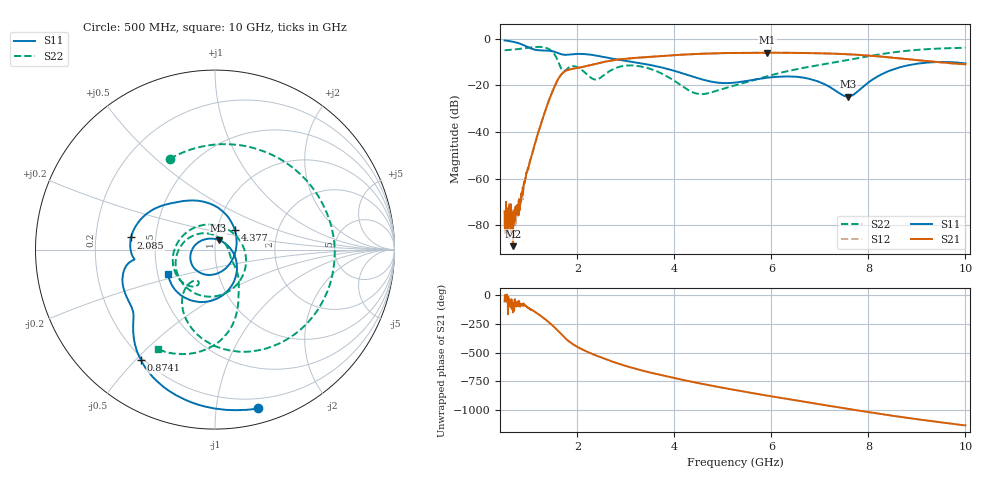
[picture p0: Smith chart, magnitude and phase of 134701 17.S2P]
!  2-Port S-parameters saved by WinCal
! VAR MeasName=S-Parameters (CALIBRATED_DATA) read from VNA (N5242A)
! VAR MeasDate=2013-7-3 16:30:44
! VAR NAME=134701 17
! VAR FILENAME=134701 17.S2P
! VAR DATE=2013-7-3 16:30:44
! VAR PHYS_PORTS=1,2
# Hz S MA R 50
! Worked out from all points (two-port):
!   1601 points, 500 MHz to 10 GHz, reference 50 ohm
!   highest |S21| = -6.01 dB at 5.915 GHz (marker M1); lowest = -88.9 dB at 672.2 MHz (marker M2)
!   |S21| within 3 dB of the highest: 2.814 GHz to 8.922 GHz (6.108 GHz wide, 104 % of centre)
!   lowest |S11| = -24.8 dB at 7.577 GHz (marker M3), VSWR 1.12, Z = 51.7 + j5.59 ohm
!   |S11| at or under -10 dB: 3.142 GHz to 9.425 GHz (6.283 GHz wide, 100 % of centre); 9.634 GHz to end of sweep
!   |S22| runs from -23.8 to -3.5 dB; largest |S21 - S12| = 0.0029
!   S11 on the Smith chart (normalised r, x): 500 MHz: 0.12, -1.30; 874.1 MHz: 0.19, -0.52; 2.085 GHz: 0.36, +0.06; 4.377 GHz: 1.22, +0.27; 10 GHz: 0.57, -0.17
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5e8  0.9171 -74.8  0.0001989 -52.0  0.0001197 -51.5  0.5646 116.6
6.721875e8  0.8623 -98.5  3.575e-05 -147.8  0.0002103 -70.3  0.5844 91.2
7.85e8  0.8037 -113.2  0.0001634 -95.1  0.0003337 -87.2  0.6021 72.9
8.740625e8  0.7412 -123.8  0.0006473 -90.7  0.0003575 -83.7  0.618 57.1
1.170938e9  0.571 -143.3  0.008142 -156.5  0.008118 -156.0  0.6682 -5.5
1.408438e9  0.5531 -157.2  0.0459 127.3  0.04596 127.1  0.6042 -69.5
1.550938e9  0.516 -167.8  0.1055 72.8  0.1052 72.7  0.4231 -112.1
1.6875e9  0.459 -172.7  0.1799 13.2  0.1796 13.0  0.2096 -123.9
1.871562e9  0.4634 -176.3  0.2233 -54.8  0.2228 -55.0  0.255 -131.3
2.085312e9  0.4728 171.8  0.2454 -108.0  0.2448 -108.0  0.2163 172.9
2.370312e9  0.4383 155.0  0.2881 -161.5  0.2875 -161.5  0.1329 67.0
2.655312e9  0.3853 140.8  0.3348 152.6  0.3346 152.5  0.1992 -32.9
3.130312e9  0.3175 121.2  0.3832 88.4  0.3825 88.3  0.2676 -118.1
3.670625e9  0.2509 93.2  0.4224 30.2  0.4214 30.2  0.1934 174.9
4.377188e9  0.1546 44.1  0.4665 -34.7  0.4669 -34.6  0.07102 74.2
5.25e9  0.1145 -45.1  0.4957 -105.3  0.4963 -105.4  0.09984 -27.7
5.915e9  0.1457 -104.0  0.5009 -154.5  0.5009 -154.6  0.1566 -42.3
6.835312e9  0.1335 -174.5  0.4903 141.3  0.4904 141.2  0.256 -58.8
7.5775e9  0.05733 70.0  0.4634 90.6  0.464 90.4  0.3492 -68.9
8.420625e9  0.2027 -57.6  0.3999 35.0  0.3995 34.9  0.4941 -84.8
9.150938e9  0.3039 -106.0  0.3357 -8.3  0.335 -8.5  0.5904 -102.2
1e10  0.2955 -152.5  0.2837 -54.3  0.2829 -54.7  0.6395 -119.8
